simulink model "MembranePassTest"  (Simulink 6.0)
settings: Solver=ode3  StartTime=0.0  StopTime=SimTime  FixedStep=1E-5  RelTol=1e-5
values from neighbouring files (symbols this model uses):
  Cmem = 1E-6*Sm*(1-b)    (= 2.826e-08)    [Constantes.m]    (also in ConstantesBck.m = 3.14e-11; ImpedanceZtissus.m = 4e-08; Ztissus.m = 4e-08; CalculCharge.m = 1)
  I0Stim = AddI    (= 0)    [WaveComp.m]    (also in WaveCompIET.m; WaveCompIETAnim.m; WaveCompIETIf.m; WaveCompIETSeul.m = Hm(i)*1E-6)
  Rcan = 6.398E3*Sm*(1-b)    (= 180.80748)    [Constantes.m]    (also in ConstantesBck.m = 0.03454; ImpedanceZtissus.m = 44; Ztissus.m = 44)
  T0Stim = i    [WaveComp.m]    (also in WaveCompIET.m; WaveCompIETAnim.m = 5; WaveCompIETIf.m; WaveCompIETSeul.m = T0Hm(i)*1E-3)
  TypeStim = 5    [WaveComp.m]    (also in WaveCompIET.m; WaveCompIETAnim.m; WaveCompIETIf.m; WaveCompIETSeul.m)
libraries: simulink x1

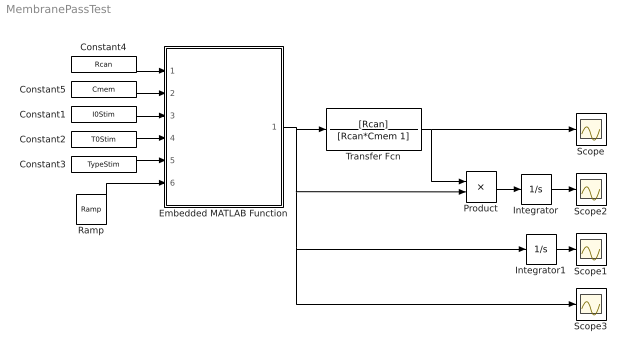
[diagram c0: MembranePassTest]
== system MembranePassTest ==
  Constant1 : Constant  Value=I0Stim
  Constant2 : Constant  Value=T0Stim
  Constant3 : Constant  Value=TypeStim
  Constant4 : Constant  Value=Rcan
  Constant5 : Constant  Value=Cmem
  Embedded MATLAB Function : Stateflow chart
  Integrator : Integrator
  Integrator1 : Integrator
  Product : Product
  Ramp : simulink/Sources/Ramp  slope=1  start=0  X0=0
  Scope{,1..3} (4 alike) : Scope
  Transfer Fcn : TransferFcn  Numerator=[Rcan]  Denominator=[Rcan*Cmem 1]
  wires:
  Product/1 -> Integrator/1
  Integrator/1 -> Scope2/1
  Constant1/1 -> Embedded MATLAB Function/3(I0Stim)
  Constant2/1 -> Embedded MATLAB Function/4(T0Stim)
  Constant3/1 -> Embedded MATLAB Function/5(TypeStim)
  Integrator1/1 -> Scope1/1
  Ramp/1 -> Embedded MATLAB Function/6(temps)
  Embedded MATLAB Function/1(Istim) -> Transfer Fcn/1, Scope3/1, Integrator1/1, Product/2
  Constant4/1 -> Embedded MATLAB Function/1(Rcan)
  Constant5/1 -> Embedded MATLAB Function/2(Cmem)
  Transfer Fcn/1 -> Scope/1, Product/1

== matlab function Embedded
MATLAB Function ==
function Istim = courant(Rcan,Cmem,I0Stim,T0Stim,TypeStim,temps)
% This block supports an embeddable subset of the MATLAB language.
% See the help menu for details. 
taum = Rcan*Cmem;
if temps <= T0Stim
    if TypeStim == 0
        Iout = I0Stim;
    elseif TypeStim == 1
        Iout = I0Stim*exp(temps/taum);
    elseif TypeStim == 2
        Iout = I0Stim*sin(pi/T0Stim*temps);
    elseif TypeStim == 3
        Iout = I0Stim*sin(pi/(2*T0Stim)*temps);
    elseif TypeStim == 4
        Iout = I0Stim*sinh(temps/taum);
    else
        Iout = I0Stim*(sin(pi/T0Stim*temps)+1/3*sin(3*pi/T0Stim*temps));
    end
else
    Iout = 0;
end
Istim = Iout;
